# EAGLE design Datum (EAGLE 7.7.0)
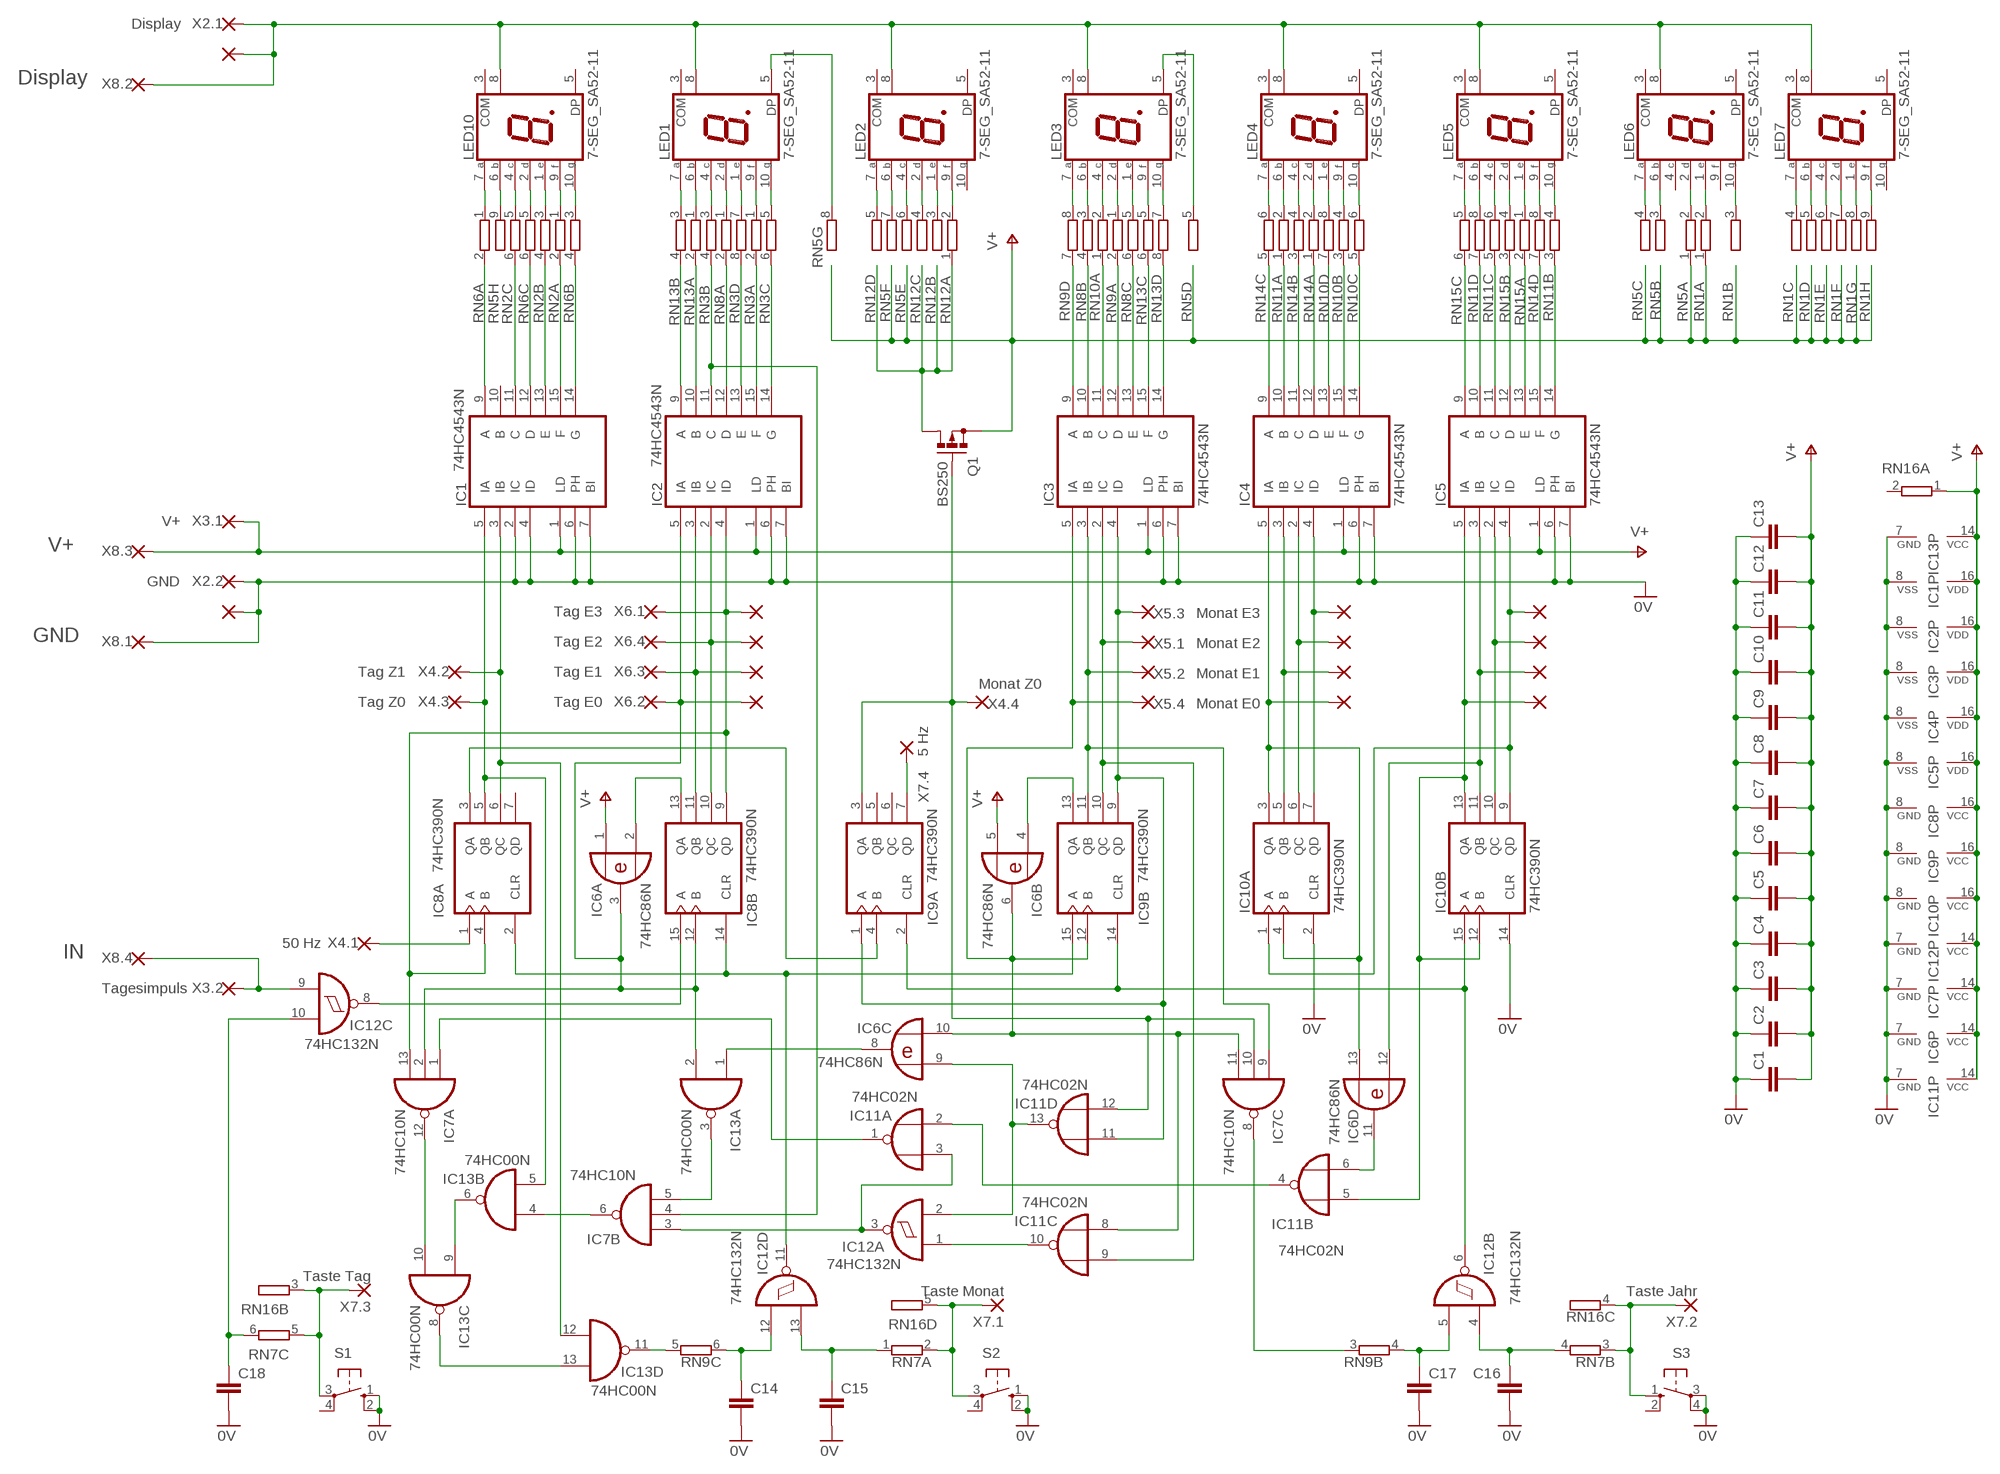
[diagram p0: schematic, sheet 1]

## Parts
102  WIREPAD1,6/0,8  [1,6/0,8]
104  WIREPAD1,6/0,8  [1,6/0,8]
111  WIREPAD1,6/0,8  [1,6/0,8]
112  WIREPAD1,6/0,8  [1,6/0,8]
113  Tag E0  WIREPAD1,6/0,8  [1,6/0,8]
114  WIREPAD1,6/0,8  [1,6/0,8]
119  WIREPAD1,6/0,8  [1,6/0,8]
120  WIREPAD1,6/0,8  [1,6/0,8]
121  WIREPAD1,6/0,8  [1,6/0,8]
122  WIREPAD1,6/0,8  [1,6/0,8]
123  WIREPAD1,6/0,8  [1,6/0,8]
124  WIREPAD1,6/0,8  [1,6/0,8]
125  WIREPAD1,6/0,8  [1,6/0,8]
126  WIREPAD1,6/0,8  [1,6/0,8]
C1  C-EU050-024X044  [C050-024X044]
C2  C-EU050-024X044  [C050-024X044]
C3  C-EU050-024X044  [C050-024X044]
C4  C-EU050-024X044  [C050-024X044]
C5  C-EU050-024X044  [C050-024X044]
C6  C-EU050-024X044  [C050-024X044]
C7  C-EU050-024X044  [C050-024X044]
C8  C-EU050-024X044  [C050-024X044]
C9  C-EU050-024X044  [C050-024X044]
C10  C-EU050-024X044  [C050-024X044]
C11  C-EU050-024X044  [C050-024X044]
C12  C-EU050-024X044  [C050-024X044]
C13  C-EU050-024X044  [C050-024X044]
C14  C-EU050-024X044  [C050-024X044]
C15  C-EU050-024X044  [C050-024X044]
C16  C-EU050-024X044  [C050-024X044]
C17  C-EU050-024X044  [C050-024X044]
C18  C-EU050-024X044  [C050-024X044]
IC1  74HC4543N  4543N  [DIL16]
IC2  74HC4543N  4543N  [DIL16]
IC3  74HC4543N  4543N  [DIL16]
IC4  74HC4543N  4543N  [DIL16]
IC5  74HC4543N  4543N  [DIL16]
IC6  74HC86N  [DIL14]
IC7  74HC10N  [DIL14]
IC8  74HC390N  [DIL16]
IC9  74HC390N  [DIL16]
IC10  74HC390N  [DIL16]
IC11  74HC02N  [DIL14]
IC12  74HC132N  [DIL14]
IC13  74HC00N  [DIL14]
LED1  7-SEG_SA52-11  [SA52-11]
LED2  7-SEG_SA52-11  [SA52-11]
LED3  7-SEG_SA52-11  [SA52-11]
LED4  7-SEG_SA52-11  [SA52-11]
LED5  7-SEG_SA52-11  [SA52-11]
LED6  7-SEG_SA52-11  [SA52-11]
LED7  7-SEG_SA52-11  [SA52-11]
LED10  7-SEG_SA52-11  [SA52-11]
Q1  BS250  [SOT54E]
RN1  GE08R  [SIL9]
RN2  E3R  [SIL6]
RN3  E4R  [SIL8]
RN5  GE08R  [SIL9]
RN6  E3R  [SIL6]
RN7  E3R  [SIL6]
RN8  E3R  [SIL6]
RN9  E4R  [SIL8]
RN10  E4R  [SIL8]
RN11  E4R  [SIL8]
RN12  GE04R  [SIL5]
RN13  E4R  [SIL8]
RN14  E4R  [SIL8]
RN15  E3R  [SIL6]
RN16  GE04R  [SIL5]
S1  10-XX  [B3F-10XX]
S2  10-XX  [B3F-10XX]
S3  10-XX  [B3F-10XX]
X2.1  Display  WIREPAD1,6/0,8  [1,6/0,8]
X2.2  GND  WIREPAD1,6/0,8  [1,6/0,8]
X3.1  V+  WIREPAD1,6/0,8  [1,6/0,8]
X3.2  Tagesimpuls  WIREPAD1,6/0,8  [1,6/0,8]
X4.1  50 Hz  WIREPAD1,6/0,8  [1,6/0,8]
X4.2  Tag Z1  WIREPAD1,6/0,8  [1,6/0,8]
X4.3  Tag Z0  WIREPAD1,6/0,8  [1,6/0,8]
X4.4  Monat Z0  WIREPAD1,6/0,8  [1,6/0,8]
X5.1  Monat E2  WIREPAD1,6/0,8  [1,6/0,8]
X5.2  Monat E1  WIREPAD1,6/0,8  [1,6/0,8]
X5.3  Monat E3  WIREPAD1,6/0,8  [1,6/0,8]
X5.4  Monat E0  WIREPAD1,6/0,8  [1,6/0,8]
X6.1  Tag E3  WIREPAD1,6/0,8  [1,6/0,8]
X6.2  Tag E0  WIREPAD1,6/0,8  [1,6/0,8]
X6.3  Tag E1  WIREPAD1,6/0,8  [1,6/0,8]
X6.4  Tag E2  WIREPAD1,6/0,8  [1,6/0,8]
X7.1  Taste Monat  WIREPAD1,6/0,8  [1,6/0,8]
X7.2  Taste Jahr  WIREPAD1,6/0,8  [1,6/0,8]
X7.3  Taste Tag  WIREPAD1,6/0,8  [1,6/0,8]
X7.4  5 Hz  WIREPAD1,6/0,8  [1,6/0,8]
X8.1  WIREPAD1,6/0,8  [1,6/0,8]
X8.2  WIREPAD1,6/0,8  [1,6/0,8]
X8.3  WIREPAD1,6/0,8  [1,6/0,8]
X8.4  WIREPAD1,6/0,8  [1,6/0,8]

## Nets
0V: 104.1(P) C1.1 C2.1 C3.1 C4.1 C5.1 C6.1 C7.1 C8.1 C9.1 C10.1 C11.1 C12.1 C13.1 C14.2 C15.2 C16.2 C17.2 C18.2 IC1.2(IC) IC1.4(ID) IC1.6(PH) IC1.7(BI) IC1.8(VSS) IC2.6(PH) IC2.7(BI) IC2.8(VSS) IC3.6(PH) IC3.7(BI) IC3.8(VSS) IC4.6(PH) IC4.7(BI) IC4.8(VSS) IC5.6(PH) IC5.7(BI) IC5.8(VSS) IC6.7(P:GND) IC7.7(P:GND) IC8.8(P:GND) IC9.8(P:GND) IC10.2(A:CLR) IC10.8(P:GND) IC10.14(B:CLR) IC11.7(P:GND) IC12.7(P:GND) IC13.7(P:GND) S1.1(S) S1.2(S1) S2.1(S) S2.2(S1) S3.3(P) S3.4(P1) X2.2.1(P) X8.1.1(P)
N$1: LED3.7(A) RN9.8
N$2: LED3.6(B) RN8.3
N$3: LED3.4(C) RN10.2
N$4: LED3.2(D) RN9.1
N$5: LED3.1(E) RN8.5
N$6: LED3.9(F) RN13.5
N$7: LED3.10(G) RN13.7
N$8: LED3.5(DP) RN5.5
N$9: LED1.5(DP) RN5.8
N$10: LED2.7(A) RN12.5
N$11: LED2.4(C) RN5.6
N$12: LED2.6(B) RN5.7
N$13: LED2.2(D) RN12.4
N$14: LED2.1(E) RN12.3
N$15: LED2.9(F) RN12.2
N$16: Q1.D RN12.1
N$17: IC6.2(A:I1) IC8.13(B:QA)
N$18: IC9.2(A:CLR) IC9.14(B:CLR) IC10.15(B:A) IC12.6(B:O)
N$19: LED6.7(A) RN5.4
N$20: IC3.9(A) RN9.7
N$21: IC3.10(B) RN8.4
N$22: LED5.4(C) RN11.6
N$23: IC3.12(D) RN9.2
N$24: IC3.13(E) RN8.6
N$25: IC3.15(F) RN13.6
N$26: IC3.14(G) RN13.8
N$27: LED4.7(A) RN14.6
N$28: LED4.6(B) RN11.2
N$29: LED4.4(C) RN14.4
N$30: LED4.2(D) RN14.2
N$31: LED4.1(E) RN10.8
N$32: LED4.9(F) RN10.4
N$33: LED4.10(G) RN10.6
N$34: LED5.7(A) RN15.5
N$35: LED5.6(B) RN11.8
N$36: IC4.10(B) RN11.1
N$37: LED5.2(D) RN15.4
N$38: LED5.1(E) RN15.1
N$39: LED5.9(F) RN14.8
N$40: LED5.10(G) RN11.4
N$41: IC5.14(G) RN11.3
N$42: IC5.15(F) RN14.7
N$43: IC5.13(E) RN15.2
N$44: IC5.12(D) RN15.3
N$45: IC2.15(F) RN3.2
N$46: IC5.10(B) RN11.7
N$47: IC5.9(A) RN15.6
N$48: IC4.14(G) RN10.5
N$49: IC4.15(F) RN10.3
N$50: IC4.13(E) RN10.7
N$51: IC4.12(D) RN14.1
N$52: IC4.11(C) RN14.3
N$54: IC4.9(A) RN14.5
N$55: LED6.6(B) RN5.3
N$56: LED6.2(D) RN5.2
N$57: LED6.1(E) RN1.2
N$58: LED6.10(G) RN1.3
N$59: LED7.7(A) RN1.4
N$60: LED7.6(B) RN1.5
N$61: LED7.4(C) RN1.6
N$62: LED7.2(D) RN1.7
N$63: LED7.1(E) RN1.8
N$64: LED7.9(F) RN1.9
N$65: IC5.11(C) RN11.5
N$66: 102.1(P) LED1.8(COM) LED2.8(COM) LED3.8(COM) LED4.8(COM) LED5.8(COM) LED6.8(COM) LED7.8(COM) LED10.8(COM) X2.1.1(P) X8.2.1(P)
N$67: 114.1(P) IC2.5(IA) IC6.3(A:O) IC7.2(A:I1) IC8.12(B:B) IC13.2(A:I1) X6.2.1(P)
N$68: IC11.2(A:I0) IC11.4(B:O)
N$69: 111.1(P) IC2.2(IC) IC8.10(B:QC) X6.4.1(P)
N$70: 113.1(P) IC2.4(ID) IC7.13(A:I2) IC8.4(A:B) IC8.9(B:QD) X6.1.1(P)
N$71: IC1.5(IA) IC8.5(A:QB) IC13.5(B:I1) X4.3.1(P)
N$72: IC1.3(IB) IC8.6(A:QC) IC13.12(D:I0) X4.2.1(P)
N$73: IC1.9(A) RN6.2
N$74: IC3.11(C) RN10.1
N$75: IC1.11(C) RN2.6
N$76: IC1.12(D) RN6.6
N$77: IC1.13(E) RN2.4
N$78: IC1.15(F) RN2.2
N$79: IC1.14(G) RN6.4
N$80: IC2.9(A) RN13.4
N$81: IC2.10(B) RN13.2
N$82: IC2.11(C) IC7.4(B:I1) RN3.4
N$83: IC2.12(D) RN8.2
N$84: IC2.13(E) RN3.8
N$86: IC2.14(G) RN3.6
N$87: LED1.10(G) RN3.5
N$88: LED1.9(F) RN3.1
N$89: LED1.1(E) RN3.7
N$90: LED1.2(D) RN8.1
N$91: LED1.4(C) RN3.3
N$92: LED1.6(B) RN13.1
N$93: LED1.7(A) RN13.3
N$94: LED10.10(G) RN6.3
N$95: LED10.9(F) RN2.1
N$96: LED10.1(E) RN2.3
N$97: LED10.2(D) RN6.5
N$98: LED10.4(C) RN2.5
N$99: LED10.6(B) RN5.9
N$100: LED10.7(A) RN6.1
N$101: IC6.4(B:I0) IC9.13(B:QA)
N$102: IC3.3(IB) IC7.9(C:I0) IC9.11(B:QB) X5.2.1(P)
N$103: IC3.2(IC) IC9.10(B:QC) IC11.9(C:I1) X5.1.1(P)
N$104: IC3.4(ID) IC9.1(A:A) IC9.9(B:QD) IC11.11(D:I0) X5.3.1(P)
N$105: 122.1(P) IC4.5(IA) IC6.13(D:I1) IC10.3(A:QA) IC10.4(A:B)
N$106: 120.1(P) IC4.3(IB) IC10.5(A:QB)
N$107: 119.1(P) IC4.2(IC) IC10.6(A:QC)
N$108: 121.1(P) IC4.4(ID) IC10.7(A:QD)
N$109: 126.1(P) IC5.5(IA) IC10.12(B:B) IC10.13(B:QA) IC11.5(B:I0)
N$110: 124.1(P) IC5.3(IB) IC6.12(D:I0) IC10.11(B:QB)
N$111: 123.1(P) IC5.2(IC) IC10.10(B:QC)
N$112: 125.1(P) IC5.4(ID) IC10.1(A:A) IC10.9(B:QD)
N$113: IC3.5(IA) IC6.6(B:O) IC6.10(C:I1) IC7.11(C:I2) IC9.12(B:B) IC11.8(C:I0) X5.4.1(P)
N$114: IC7.3(B:I0) IC11.3(A:I1) IC12.3(A:O)
N$115: IC7.5(B:I2) IC13.3(A:O)
N$116: IC7.1(A:I0) IC11.1(A:O)
N$117: IC6.8(C:O) IC13.1(A:I0)
N$118: IC7.12(A:O) IC13.10(C:I1)
N$119: IC13.6(B:O) IC13.9(C:I0)
N$120: IC7.6(B:O) IC13.4(B:I0)
N$121: IC13.8(C:O) IC13.13(D:I1)
N$122: IC8.2(A:CLR) IC8.14(B:CLR) IC9.15(B:A) IC12.11(D:O)
N$123: IC6.9(C:I0) IC11.13(D:O) IC12.2(A:I1)
N$124: IC11.10(C:O) IC12.1(A:I0)
N$125: IC12.9(C:I0) X3.2.1(P) X8.4.1(P)
N$126: 112.1(P) IC2.3(IB) IC8.11(B:QB) X6.3.1(P)
N$127: IC7.10(C:I1) IC9.3(A:QA) IC11.12(D:I1) Q1.G X4.4.1(P)
N$128: IC8.15(B:A) IC12.8(C:O)
N$129: IC6.11(D:O) IC11.6(B:I1)
N$131: IC13.11(D:O) RN9.5
N$132: C14.1 IC12.12(D:I0) RN9.6
N$133: RN7.2 RN16.5 S2.3(P) X7.1.1(P)
N$134: C15.1 IC12.13(D:I1) RN7.1
N$135: C17.1 IC12.5(B:I1) RN9.4
N$136: IC7.8(C:O) RN9.3
N$137: RN7.3 RN16.4 S3.1(S) X7.2.1(P)
N$138: C16.1 IC12.4(B:I0) RN7.4
N$139: C18.1 IC12.10(C:I1) RN7.6
N$140: RN7.5 RN16.3 S1.3(P) X7.3.1(P)
N$143: IC8.1(A:A) X4.1.1(P)
N$144: IC9.7(A:QD) X7.4.1(P)
N$145: IC8.3(A:QA) IC9.4(A:B)
V+: C1.2 C2.2 C3.2 C4.2 C5.2 C6.2 C7.2 C8.2 C9.2 C10.2 C11.2 C12.2 C13.2 IC1.1(LD) IC1.16(VDD) IC2.1(LD) IC2.16(VDD) IC3.1(LD) IC3.16(VDD) IC4.1(LD) IC4.16(VDD) IC5.1(LD) IC5.16(VDD) IC6.1(A:I0) IC6.5(B:I1) IC6.14(P:VCC) IC7.14(P:VCC) IC8.16(P:VCC) IC9.16(P:VCC) IC10.16(P:VCC) IC11.14(P:VCC) IC12.14(P:VCC) IC13.14(P:VCC) Q1.S RN1.1 RN5.1 RN16.1 X3.1.1(P) X8.3.1(P)
Unconnected: IC1.10(B) IC8.7(A:QD) IC9.5(A:QB) IC9.6(A:QC) LED1.3(COM) LED2.3(COM) LED2.5(DP) LED2.10(G) LED3.3(COM) LED4.3(COM) LED4.5(DP) LED5.3(COM) LED5.5(DP) LED6.3(COM) LED6.4(C) LED6.5(DP) LED6.9(F) LED7.3(COM) LED7.5(DP) LED7.10(G) LED10.3(COM) LED10.5(DP) RN16.2 S1.4(P1) S2.4(P1) S3.2(S1)

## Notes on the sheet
- Display
- V+
- GND
- IN

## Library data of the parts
102 104 111-114 119-126 X2.1 X2.2 X3.1 X3.2 X4.1-X4.4 X5.1-X5.4 X6.1-X6.4 X7.1-X7.4 X8.1-X8.4 = wirepad:WIREPAD: Wire PAD connect wire on PCB
C1-C18 = rclxrund:C-EU: CAPACITOR, European symbol; SPICEPREFIX: C
IC1-IC5 = 45xxrund:4543: BCD to 7-segment LCD DECODER
IC6 = 74xx-eu:74*86: Quad 2-input EXCLUSIVE-OR (XOR) gate
IC7 = 74xx-eu:74*10: Triple 3-input NAND gate
IC8-IC10 = 74xx-eu:74*390: Dual 4-bit decade and binary COUNTER
IC11 = 74xx-eu:74*02: Quad 2-input NOR gate
IC12 = 74xx-eu:74*132: Quad 2-input NAND schmitt trigger
IC13 = 74xx-eu:74*00: Quad 2-input NAND gate
LED1-LED7 LED10 = display-kingbrightyx:7-SEG_: Kingbright 14.2mm (0.56 INCH) SINGLE DIGIT NUMERIC DUISPLAY Source: SA56-11EWA(Ver1189471036.pdf; OC_FARNELL: unknown; OC_NEWARK: unknown
Q1 = transistor-small-signal:BS250: P-CHANNEL MOS FET
RN1 RN5 = resistor-silxrund:GE08R: SIL RESISTOR; OC_FARNELL: unknown; OC_NEWARK: unknown
RN2 RN6-RN8 RN15 = resistor-silxrund:E3R: SIL RESISTOR; OC_FARNELL: unknown; OC_NEWARK: unknown
RN3 RN9-RN11 RN13 RN14 = resistor-silxrund:E4R: SIL RESISTOR; OC_FARNELL: unknown; OC_NEWARK: unknown
RN12 RN16 = resistor-silxrund:GE04R: SIL RESISTOR; OC_FARNELL: unknown; OC_NEWARK: unknown
S1-S3 = switch-omronxrund:10-XX: OMRON SWITCH; MPN: B3F-1000; OC_FARNELL: 176432; OC_NEWARK: 36M3542

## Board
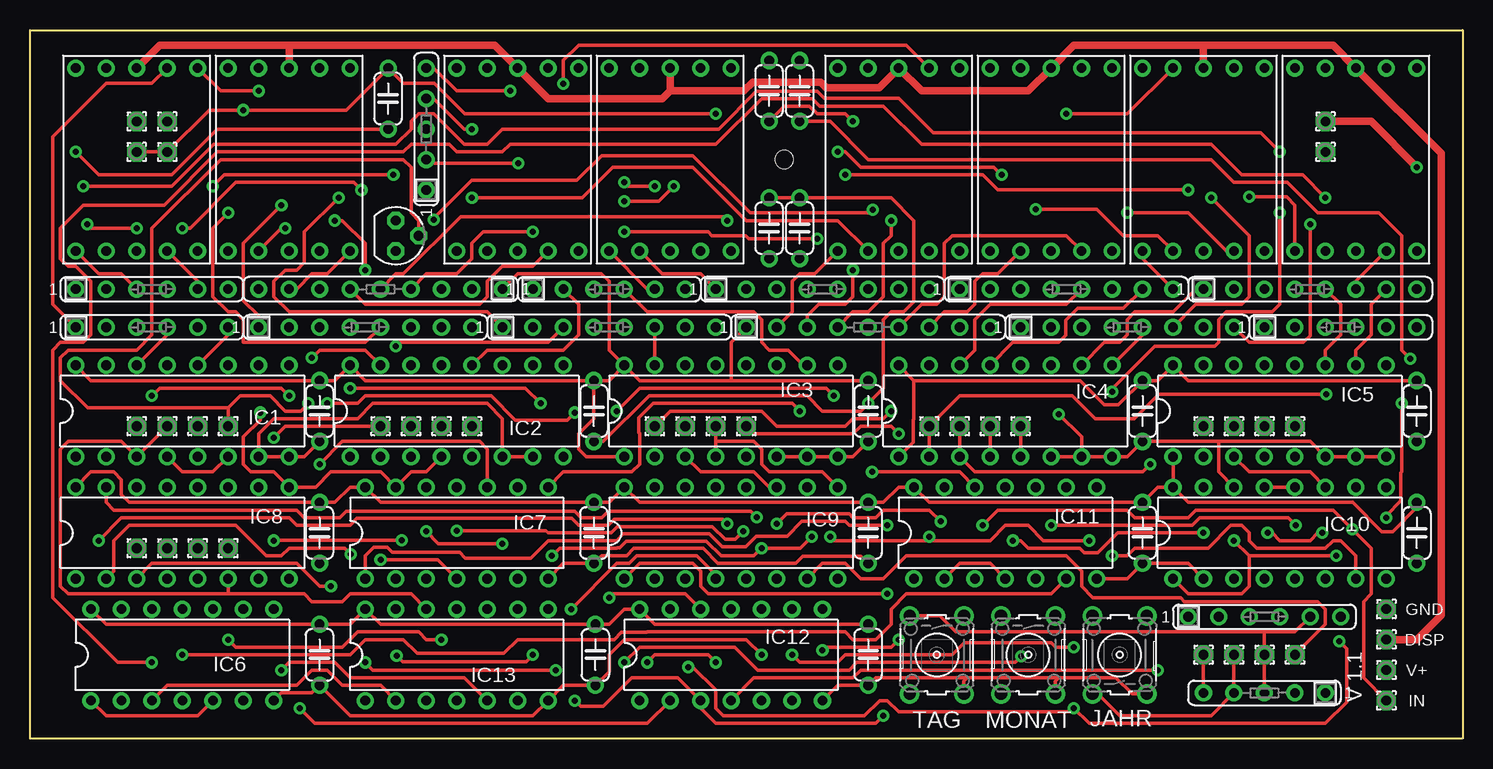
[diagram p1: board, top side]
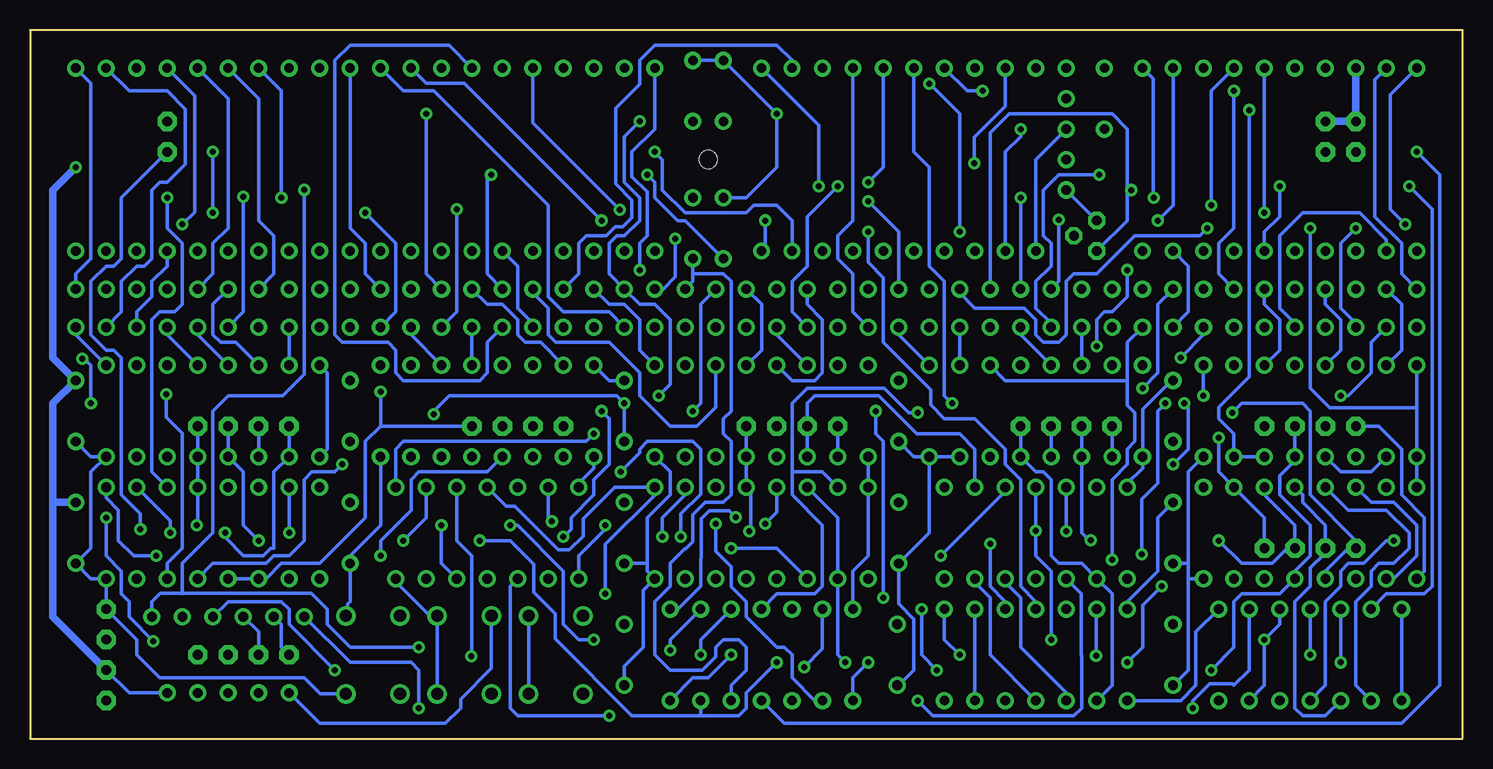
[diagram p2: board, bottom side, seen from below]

Size 119.38 x 59.05 mm. Coordinates in mm from the lower left corner, seen from the top.
Outline: 0,0 0,59.05 119.38,59.05 119.38,0 0,0
Copper layers (1*16): Top 0.035mm / dielectric 1.5mm / Bottom 0.035mm
Design rules "12mil *": minimum track width 12mil, minimum drill 0.5mm, track to track 12mil, track to pad 14mil, pad to pad 16mil, via to via 16mil, smd to smd 6mil, copper to edge 35mil, drill to drill 12mil, minimum pad ring 12mil, minimum via ring 10mil, stop-mask expansion 4mil, vias tented up to drill 0mil, thermal gap 10mil
Holes 1.5 mm at 62.87,48.26

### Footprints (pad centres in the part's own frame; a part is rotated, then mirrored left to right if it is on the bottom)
1,6/0,8 = drill 0.813 pad 1.6 octagon: 1 0,0
C050-024X044 = drill 0.813: 1 -2.54,0; 2 2.54,0
DIL16 = drill 0.813: 1 -8.89,-3.81; 2 -6.35,-3.81; 3 -3.81,-3.81; 4 -1.27,-3.81; 5 1.27,-3.81; 6 3.81,-3.81; 7 6.35,-3.81; 8 8.89,-3.81; 9 8.89,3.81; 10 6.35,3.81; 11 3.81,3.81; 12 1.27,3.81; 13 -1.27,3.81; 14 -3.81,3.81; 15 -6.35,3.81; 16 -8.89,3.81
DIL14 = drill 0.813: 1 -7.62,-3.81; 2 -5.08,-3.81; 3 -2.54,-3.81; 4 0,-3.81; 5 2.54,-3.81; 6 5.08,-3.81; 7 7.62,-3.81; 8 7.62,3.81; 9 5.08,3.81; 10 2.54,3.81; 11 0,3.81; 12 -2.54,3.81; 13 -5.08,3.81; 14 -7.62,3.81
SA52-11 = drill 0.8: 1 -5.08,-7.62; 2 -2.54,-7.62; 3 0,-7.62; 4 2.54,-7.62; 5 5.08,-7.62; 6 5.08,7.62; 7 2.54,7.62; 8 0,7.62; 9 -2.54,7.62; 10 -5.08,7.62
SOT54E = drill 0.813 octagon: D -1.27,0; G 0,1.905; S 1.27,0
SIL9 = drill 0.813: 1 -10.16,0; 2 -7.62,0; 3 -5.08,0; 4 -2.54,0; 5 0,0; 6 2.54,0; 7 5.08,0; 8 7.62,0; 9 10.16,0
SIL6 = drill 0.813: 1 -6.35,0; 2 -3.81,0; 3 -1.27,0; 4 1.27,0; 5 3.81,0; 6 6.35,0
SIL8 = drill 0.813: 1 -8.89,0; 2 -6.35,0; 3 -3.81,0; 4 -1.27,0; 5 1.27,0; 6 3.81,0; 7 6.35,0; 8 8.89,0
SIL5 = drill 0.813: 1 -5.08,0; 2 -2.54,0; 3 0,0; 4 2.54,0; 5 5.08,0
B3F-10XX = drill 1.016: 1 -3.251,2.261; 2 3.251,2.261; 3 -3.251,-2.261; 4 3.251,-2.261

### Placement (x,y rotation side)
102  11.43,51.44 0 top
104  11.43,48.9 0 top
111  29.21,26.04 0 top
112  31.75,26.04 0 top
113  34.29,26.04 0 top
114  36.83,26.04 0 top
119  74.93,26.04 0 top
120  77.47,26.04 0 top
121  80.01,26.04 0 top
122  82.55,26.04 0 top
123  97.79,26.04 0 top
124  100.33,26.04 0 top
125  102.87,26.04 0 top
126  105.41,26.04 0 top
C1  115.57,27.3 90 top
C2  24.13,27.3 90 top
C3  46.99,27.3 90 top
C4  69.85,27.3 90 top
C5  92.71,27.3 90 top
C6  115.57,17.14 90 top
C7  24.13,17.14 90 top
C8  69.85,6.99 90 top
C9  24.13,6.99 90 top
C10  92.71,17.14 90 top
C11  69.85,17.14 90 top
C12  46.99,17.14 90 top
C13  47.12,6.99 90 top
C14  61.59,53.98 90 top
C15  64.14,53.98 90 top
C16  29.84,53.34 90 top
C17  64.14,42.55 90 top
C18  61.59,42.55 90 top
IC1  12.7,27.3 0 top
IC2  35.56,27.3 0 top
IC3  58.42,27.3 0 top
IC4  81.28,27.3 0 top
IC5  104.14,27.3 0 top
IC6  12.7,6.99 0 top
IC7  35.56,17.14 0 top
IC8  12.7,17.14 0 top
IC9  58.42,17.14 0 top
IC10  104.14,17.14 0 top
IC11  81.28,17.14 0 top
IC12  58.42,6.99 0 top
IC13  35.56,6.99 0 top
LED1  21.59,48.26 0 top
LED2  40.64,48.26 0 top
LED3  53.34,48.26 0 top
LED4  97.79,48.26 0 top
LED5  110.49,48.26 0 top
LED6  72.39,48.26 0 top
LED7  85.09,48.26 0 top
LED10  8.89,48.26 0 top
Q1  30.48,41.91 270 top
RN1  69.85,34.29 0 top
RN2  10.16,37.47 0 top
RN3  27.94,34.29 0 top
RN5  29.21,37.47 180 top
RN6  10.16,34.29 0 top
RN7  102.87,10.16 0 top
RN8  48.26,37.47 0 top
RN9  66.04,37.47 0 top
RN10  86.36,37.47 0 top
RN11  106.68,37.47 0 top
RN12  33.02,50.8 90 top
RN13  48.26,34.29 0 top
RN14  91.44,34.29 0 top
RN15  109.22,34.29 0 top
RN16  102.87,3.81 180 top
S1  75.56,6.99 270 top
S2  83.19,6.99 270 top
S3  90.81,6.99 90 top
X2.1  8.89,51.44 0 top
X2.2  8.89,48.9 0 top
X3.1  107.95,51.44 0 top
X3.2  107.95,48.9 0 top
X4.1  8.89,26.04 0 top
X4.2  11.43,26.04 0 top
X4.3  13.97,26.04 0 top
X4.4  16.51,26.04 0 top
X5.1  52.07,26.04 0 top
X5.2  54.61,26.04 0 top
X5.3  57.15,26.04 0 top
X5.4  59.69,26.04 0 top
X6.1  8.89,15.88 0 top
X6.2  11.43,15.88 0 top
X6.3  13.97,15.88 0 top
X6.4  16.51,15.88 0 top
X7.1  97.79,6.99 0 top
X7.2  100.33,6.99 0 top
X7.3  102.87,6.99 0 top
X7.4  105.41,6.99 0 top
X8.1  113.03,10.79 0 top
X8.2  113.03,8.26 0 top
X8.3  113.03,5.71 0 top
X8.4  113.03,3.17 0 top

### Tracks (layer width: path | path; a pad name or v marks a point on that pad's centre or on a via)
0V  (via drill 0.5)
  Top 0.305: IC5.8 IC5.7 IC5.6 106.68,24.77 99.06,24.77 | IC4.7 IC4.6 | IC4.7 IC4.8 91.44,23.5 C5.1 99.06,24.77 | IC10.14 99.06,22.23 99.06,24.77 | IC3.6 IC3.7 IC3.8 68.58,23.5 C4.1 | IC12.7 67.31,4.45 C8.1 70.48,5.08 78.11,5.08 | IC11.7 91.44,13.34 C10.1 96.52,14.61 IC10.2 | 85.72,5.08 90.49,5.08 91.83,3.73 S3.3 | S2.2 85.45,4.8 85.72,5.08 | C18.2 C17.2 71.75,45.09 73.66,43.18 73.66,36.42 72.8,35.56 71.75,35.56 71.12,34.92 71.12,29.21 v69.85,27.94 69.22,27.3 66.04,27.3 64.77,28.57 51.6,28.57 47.79,24.77 C3.1 | IC7.7 44.45,14.61 C12.1 47.62,15.24 49.71,15.24 50.32,15.85 56.11,15.85 57.33,14.63 63.82,14.63 64.4,15.21 69.24,15.21 C11.1 | IC2.7 IC2.6 39.37,26.67 38.1,27.94 28.57,27.94 27.3,26.67 20.32,26.67 19.05,25.4 IC1.7 IC1.8 22.86,23.5 C2.1 | IC6.7 20.95,3.81 23.5,3.81 C9.1 26.67,1.91 41.91,1.91 IC13.7 44.45,4.45 C13.1 48.26,5.59 48.26,6.99 49.53,8.26 59.69,8.26 v60.96,6.99 | IC1.4 12.7,22.23 15.24,22.23 IC1.6 | v85.72,27.05 87.63,25.14 IC4.7 | 85.72,5.08 78.11,5.08 | S1.2 77.83,4.8 78.11,5.08 | v57.15,52.07 36.22,52.07 33.68,54.61 31.11,54.61 C16.2 26.35,52.39 v17.78,52.39 14.92,52.39 104.1 X2.2.1
  Bottom 0.305: 67.94,14.61 67.94,13.97 IC9.8 68.26,12.38 68.26,7.62 69.85,6.03 C8.1 | C11.1 67.94,14.61 | IC3.8 66.04,22.23 66.04,20.32 67.94,18.41 67.94,14.61 | IC11.7 88.9,13.06 86.08,10.24 S2.1 S2.2 | S3.4 92.91,11.23 92.71,11.43 C10.1 92.71,15.24 90.17,17.78 IC4.8 | IC2.7 IC2.8 | C3.1 45.72,23.5 IC2.8 | IC2.8 44.45,17.14 C12.1 46.99,11.24 45.72,9.97 45.72,5.71 46.99,4.45 C13.1 | 22.86,13.34 IC8.8 | 22.86,13.34 22.86,5.71 C9.1 | IC1.6 IC1.7 19.05,25.4 20.32,26.67 20.32,27.62 17.78,30.16 v17.78,52.39 | 22.86,14.61 22.86,22.23 IC1.8 | IC12.7 64.14,5.08 62.87,5.08 v60.96,6.99 | IC1.4 10.16,22.23 7.62,22.23 IC1.2 | C1.1 114.3,23.5 IC5.8 114.3,22.23 114.3,15.88 C6.1 114.3,13.34 IC10.8 X8.1.1 110.49,8.26 110.49,6.99 108.58,5.08 96.52,5.08 95.17,3.73 S3.3 | C4.1 v69.85,27.94 70.48,28.57 84.45,28.57 85.72,27.3 v85.72,27.05 | S1.1 S1.2 | 22.86,14.61 22.86,13.34 | C7.1 22.86,14.61 | C15.2 C14.2 v57.15,52.07 57.15,47.62 59.69,45.09 C18.2
N$1
  Bottom 0.305: RN9.8 73.66,38.73 73.66,41.27 73.03,41.91 71.37,41.91 70.61,42.67 69.98,42.67 69.96,42.66 69.22,43.41 69.22,44.86 70.58,46.22 70.58,52.55 68.58,54.55 68.58,56.52 67.31,57.78 57.15,57.78 55.88,56.52 LED3.7
N$2  (via drill 0.5)
  Top 0.305: v53.66,46.04 52.39,44.77 v49.53,44.77
  Bottom 0.305: v53.66,46.04 53.66,51.12 LED3.6 | v49.53,44.77 46.99,42.23 RN8.3
N$3  (via drill 0.5)
  Top 0.305: v67.31,48.9 67.94,48.9 69.22,47.62 80.33,47.62 v80.96,46.99
  Bottom 0.305: v67.31,48.9 66.67,48.26 66.67,45.72 64.77,43.81 59.69,43.81 59.05,44.45 57.15,44.45 55.88,43.18 LED3.4 | v80.96,46.99 81.28,46.67 81.28,38.73 RN10.2
N$4
  Top 0.305: LED3.2 52.7,38.73 55.88,38.73 RN9.1
N$5
  Top 0.305: LED3.1 51.44,37.47 RN8.5
N$6
  Bottom 0.305: LED3.9 50.8,43.18 52.07,41.91 52.07,40.01 50.8,38.73 50.8,35.56 RN13.5
N$7  (via drill 0.5)
  Top 0.305: v49.53,46.35 49.85,46.04 v52.07,46.04
  Bottom 0.305: v49.53,46.35 48.26,47.62 LED3.10 | v52.07,46.04 54.61,43.5 54.61,39.37 55.88,38.1 55.88,35.56 RN13.7
N$8  (via drill 0.5)
  Top 0.305: v58.1,43.18 57.78,43.5 35.88,43.5 31.11,38.73 30.48,38.73 RN5.5
  Bottom 0.305: LED3.5 58.1,40.96 v58.1,43.18
N$9
  Top 0.305: LED1.5 24.77,38.73 23.5,38.73 22.23,37.47 RN5.8
N$10  (via drill 0.5)
  Top 0.305: RN12.5 33.66,55.88 35.56,53.98 v40.01,53.98
  Bottom 0.305: LED2.7 41.27,53.98 v40.01,53.98
N$11
  Top 0.305: LED2.4 41.91,39.37 39.37,39.37 38.1,38.1 38.1,36.83 37.47,36.2 27.94,36.2 RN5.6
N$12  (via drill 0.5)
  Top 0.305: v42.55,27.94 41.27,29.21 v26.67,29.21
  Bottom 0.305: LED2.6 45.72,48.9 44.45,47.62 44.45,39.37 43.18,38.1 43.18,28.57 v42.55,27.94 | v26.67,29.21 25.4,30.48 25.4,36.2 RN5.7
N$13  (via drill 0.5)
  Top 0.305: v36.83,50.8 36.2,50.8 33.66,53.34 RN12.4
  Bottom 0.305: LED2.2 38.1,48.9 36.83,50.16 v36.83,50.8
N$14
  Bottom 0.305: LED2.1 35.56,48.26 RN12.3
N$15  (via drill 0.5)
  Top 0.305: v40.7,47.94 33.34,47.94 RN12.2
  Bottom 0.305: LED2.9 38.1,52.7 40.7,50.1 v40.7,47.94
N$16
  Bottom 0.305: RN12.1 Q1.D
N$17
  Bottom 0.305: IC6.2 8.89,4.45 8.89,11.43 7.62,12.7 7.62,13.97 6.99,14.61 5.71,14.61 4.45,15.88 4.45,17.14 6.35,19.05 9.53,19.05 IC8.13
N$18  (via drill 0.5)
  Top 0.305: v51.44,6.35 52.07,6.99 56.52,6.99 v57.15,6.35 | v81.92,16.51 82.55,16.51 83.19,15.88 87.47,15.88 87.85,15.5 89,15.5 90.64,17.14 v97.79,17.14
  Bottom 0.305: 63.5,1.91 60.33,1.91 59.69,2.54 59.69,3.81 v57.15,6.35 | IC9.14 52.07,18.41 IC9.2 52.07,6.99 v51.44,6.35 | v97.79,17.14 IC10.15 | 63.5,1.91 69.22,1.91 75.63,8.32 75.63,10.4 77.42,12.2 77.42,14.55 79.38,16.51 v81.92,16.51 | IC12.6 63.5,1.91
N$19  (via drill 0.5)
  Top 0.305: LED6.7 73.03,57.78 45.72,57.78 44.45,56.52 v44.45,54.58 | v41.91,42.23 37.78,42.23 36.83,41.27 36.83,40.01 35.56,38.73 33.02,38.73 RN5.4
  Bottom 0.305: v41.91,42.23 41.91,52.07 44.45,54.61 v44.45,54.58
N$20
  Bottom 0.305: IC3.9 68.58,32.38 68.58,34.92 69.85,36.2 71.12,36.2 RN9.7
N$21
  Top 0.305: RN8.4 51.44,35.56 60.33,35.56 60.96,34.92 60.96,33.02 61.59,32.38 63.18,32.38 64.45,31.11 IC3.10
N$22
  Top 0.305: LED5.4 110.49,38.1 RN11.6
N$23
  Bottom 0.305: IC3.12 58.42,32.38 58.42,36.2 RN9.2
N$24
  Bottom 0.305: RN8.6 54.61,36.2 53.34,34.92 53.34,30.48 53.98,29.84 55.88,29.84 IC3.13
N$25
  Top 0.305: RN13.6 IC3.15
N$26
  Bottom 0.305: IC3.14 57.15,33.66 RN13.8
N$27  (via drill 0.5)
  Top 0.305: RN14.6 97.16,36.2 100.97,36.2 101.6,36.83 101.6,41.91 v98.42,45.09
  Bottom 0.305: v98.42,45.09 98.42,53.98 LED4.7
N$28
  Bottom 0.305: RN11.2 99.06,38.73 99.06,41.91 100.33,43.18 100.33,53.34 LED4.6
N$29  (via drill 0.5)
  Top 0.305: v91.44,43.81 96.52,43.81 99.69,40.64 LED4.4
  Bottom 0.305: v91.44,43.81 88.9,41.27 88.9,35.56 RN14.4
N$30  (via drill 0.5)
  Top 0.305: LED4.2 93.98,41.91 91.12,41.91 88.9,44.13 v83.82,44.13
  Bottom 0.305: v83.82,44.13 83.82,35.56 RN14.2
N$31
  Top 0.305: RN10.8 92.71,40.01 LED4.1
N$32  (via drill 0.5)
  Top 0.305: LED4.9 91.44,52.07 v86.36,52.07
  Bottom 0.305: v86.36,52.07 86.36,38.73 RN10.4
N$33
  Bottom 0.305: LED4.10 92.71,42.55 91.44,41.27 91.44,38.73 RN10.6
N$34
  Bottom 0.305: LED5.7 111.12,53.98 107.95,53.98 106.43,52.45 106.43,47.88 107.95,46.35 108.58,46.35 109.22,45.72 109.22,40.01 109.86,39.37 110.49,39.37 111.76,38.1 111.76,35.56 RN15.5
N$35
  Bottom 0.305: LED5.6 114.3,54.61 114.3,40.01 115.57,38.73 RN11.8
N$36
  Top 0.305: IC4.10 89.53,33.02 90.81,33.02 91.44,33.66 91.44,34.92 92.08,35.56 95.25,35.56 97.16,37.47 RN11.1
N$37
  Bottom 0.305: RN15.4 110.49,35.56 109.22,36.83 109.22,38.1 107.95,39.37 LED5.2
N$38  (via drill 0.5)
  Top 0.305: LED5.1 105.41,44.45 104.71,45.15 v101.6,45.15
  Bottom 0.305: v101.6,45.15 101.6,35.56 RN15.1
N$39  (via drill 0.5)
  Top 0.305: v106.68,42.86 106.68,33.59 106.11,33.02 101.6,33.02 RN14.8
  Bottom 0.305: v106.68,42.86 105.66,43.88 105.66,53.59 LED5.9
N$40
  Bottom 0.305: RN11.4 104.14,38.73 104.14,41.27 102.87,42.55 102.87,53.34 LED5.10
N$41
  Bottom 0.305: IC5.14 102.23,33.02 103.5,33.02 104.14,33.66 104.14,36.2 RN11.3
N$42
  Bottom 0.305: RN14.7 IC5.15
N$43
  Bottom 0.305: IC5.13 105.41,33.66 RN15.2
N$44
  Bottom 0.305: IC5.12 107.95,33.66 RN15.3
N$45  (via drill 0.5)
  Top 0.305: IC2.15 27.94,32.38 24.13,32.38 v23.5,31.75
  Bottom 0.305: v23.5,31.75 21.59,33.66 RN3.2
N$46
  Top 0.305: IC5.10 110.49,32.38 111.76,33.66 111.76,36.2 RN11.7
N$47
  Bottom 0.305: IC5.9 115.57,33.66 RN15.6
N$48
  Top 0.305: IC4.14 78.74,32.38 78.74,34.92 80.01,36.2 86.36,36.2 RN10.5
N$49
  Bottom 0.305: IC4.15 76.83,33.02 78.11,33.02 78.74,33.66 78.74,34.92 80.01,36.2 81.28,36.2 RN10.3
N$50
  Top 0.305: IC4.13 81.92,33.02 85.72,33.02 86.31,33.6 86.31,34.87 87.31,35.88 91.12,35.88 RN10.7
N$51
  Bottom 0.305: RN14.1 IC4.12
N$52
  Bottom 0.305: IC4.11 87.63,33.66 RN14.3
N$54
  Top 0.305: IC4.9 92.71,33.66 RN14.5
N$55  (via drill 0.5)
  Top 0.305: v70.23,44.07 69.98,43.81 60.01,43.81 55.24,48.58 47.62,48.58 45.56,46.51 36.8,46.51 33.66,43.37 v33.66,43.24
  Bottom 0.305: LED6.6 77.47,51.31 v70.23,44.07 | v33.66,43.24 33.66,38.1 RN5.3
N$56  (via drill 0.5)
  Top 0.305: LED6.2 67.31,43.18 59.69,43.18 55.24,47.62 48.58,47.62 46.04,45.09 v36.83,45.09
  Bottom 0.305: RN5.2 v36.83,45.09
N$57
  Top 0.305: LED6.1 65.41,38.73 64.14,38.73 63.5,38.1 63.5,35.56 RN1.2
N$58  (via drill 0.5)
  Top 0.305: RN1.3 64.77,35.24 65.72,36.2 67.94,36.2 68.58,36.83 v68.58,39.05
  Bottom 0.305: LED6.10 67.31,50.8 69.22,48.9 69.22,46.83 67.94,45.56 67.94,41.91 68.58,41.27 v68.58,39.05
N$59  (via drill 0.5)
  Top 0.305: v71.75,43.18 71.75,41.91 71.12,41.27 71.12,36.83 69.85,35.56 68.58,35.56 RN1.4
  Bottom 0.305: LED7.7 86.36,54.61 83.19,54.61 v71.75,43.18
N$60
  Bottom 0.305: LED7.6 88.27,53.98 85.72,53.98 76.2,44.45 76.2,36.83 74.93,35.56 71.12,35.56 RN1.5
N$61
  Top 0.305: LED7.4 86.36,41.91 76.83,41.91 76.2,41.27 76.2,36.83 75.56,36.2 74.3,36.2 RN1.6
N$62
  Top 0.305: LED7.2 80.64,38.73 79.38,38.73 78.74,38.1 78.74,36.2 78.11,35.56 76.2,35.56 RN1.7
N$63
  Bottom 0.305: LED7.1 78.74,39.37 78.74,35.88 77.47,34.61 RN1.8
N$64
  Bottom 0.305: LED7.9 84.45,57.78 92.71,57.78 93.98,56.52 93.98,33.66 93.34,33.02 89.53,33.02 88.9,32.38 88.9,30.48 88.27,29.84 81.92,29.84 81.28,30.48 81.28,33.02 RN1.9
N$65
  Top 0.305: IC5.11 107.95,32.38 109.22,33.66 109.22,36.2 RN11.5
N$66
  Top 0.61: X8.2.1 115.57,8.26 117.6,10.29 117.6,48.77 LED5.8 108.58,57.78 97.79,57.78 | 97.79,57.78 87,57.78 LED7.8 83.19,53.98 74.3,53.98 LED6.8 70.77,54.26 66.35,54.26 65.9,54.71 60.21,54.71 59.47,53.98 53.34,53.98 | LED4.8 97.79,57.78 | 53.34,53.98 52.7,53.34 43.18,53.34 LED2.8 38.73,57.78 21.59,57.78 | 53.34,53.98 LED3.8 | 21.59,57.78 10.79,57.78 LED10.8 | LED1.8 21.59,57.78
  Bottom 0.61: LED10.8 X2.1.1 102.1
N$67
  Top 0.305: IC13.2 29.21,4.45 26.04,4.45 24.77,5.71 23.5,5.71 22.23,4.45 11.43,4.45 IC6.3
  Bottom 0.305: 114.1 IC2.5 35.56,22.23 34.92,22.23 34.29,21.59 34.29,15.24 33.66,14.61 31.75,14.61 IC7.2 29.21,12.06 29.21,4.45 IC13.2 | IC8.12 13.34,20.32 13.34,19.68 11.43,17.78 X6.2.1 11.43,15.47 12.68,14.22 12.68,13.99 12.7,13.97 12.7,12.7 13.97,11.43 13.97,2.54 13.34,1.91 11.43,1.91 IC6.3
N$68
  Top 0.305: IC11.2 77.47,14.61 80.01,14.61 IC11.4
N$69  (via drill 0.5)
  Top 0.305: v20.32,25.08 21.27,26.04 111.1
  Bottom 0.305: v20.32,25.08 20.32,22.23 IC8.10 16.51,18.41 X6.4.1 | 111.1 IC2.2
N$70  (via drill 0.5)
  Top 0.305: IC2.4 33.02,22.23 31.75,22.23 IC7.13 29.21,22.23 25.08,22.23 23.81,20.95 IC8.9 20.32,22.23 18.41,22.23 17.78,22.86 17.78,25.15 19.18,26.54 v19.18,27.18
  Bottom 0.305: IC2.4 113.1 | v19.18,27.18 18.41,27.94 13.34,27.94 12.7,27.3 12.7,20.32 8.89,16.51 X6.1.1 9.53,15.88 11.43,13.97 IC8.4
N$71  (via drill 0.5)
  Top 0.305: IC13.5 36.2,5.08 26.67,5.08 25.4,6.35 21.59,6.35 v20.95,5.71
  Bottom 0.305: v20.95,5.71 19.05,7.62 19.05,11.43 18.41,12.06 15.24,12.06 IC8.5 13.97,13.97 12.7,15.24 12.7,17.78 15.24,20.32 15.24,21.91 13.97,23.18 IC1.5 X4.3.1
N$72
  Top 0.305: X4.2.1 IC1.3 7.62,24.77 3.17,24.77 2.54,24.13 2.54,12.7 3.17,12.06 16.51,12.06 | 16.51,12.06 IC8.6 | 16.51,12.06 22.86,12.06 23.5,11.43 26.04,11.43 26.67,12.06 31.75,12.06 IC13.12
N$73  (via drill 0.5)
  Top 0.305: v21.59,28.57 20.95,29.21 10.79,29.21 v10.16,28.57
  Bottom 0.305: RN6.2 7.62,33.02 7.62,30.48 9.53,28.57 v10.16,28.57 | IC1.9 v21.59,28.57
N$74
  Bottom 0.305: IC3.11 62.23,27.62 63.82,26.04 66.04,26.04 68.58,28.57 68.58,30.48 71.12,33.02 75.56,33.02 76.2,33.66 76.2,35.88 77.47,37.15 RN10.1
N$75
  Bottom 0.305: IC1.11 15.24,32.38 15.24,34.92 16.51,36.2 RN2.6
N$76
  Top 0.305: IC1.12 16.51,33.66 RN6.6
N$77
  Bottom 0.305: IC1.13 10.16,32.38 10.16,34.92 11.43,36.2 RN2.4
N$78
  Bottom 0.305: IC1.15 5.08,32.38 5.08,36.2 RN2.2
N$79
  Top 0.305: IC1.14 11.43,33.66 RN6.4
N$80
  Bottom 0.305: IC2.9 46.99,33.66 RN13.4
N$81
  Bottom 0.305: RN13.2 IC2.10
N$82  (via drill 0.5)
  Top 0.305: IC7.4 33.97,14.92 v29.21,14.92
  Bottom 0.305: v29.21,14.92 29.21,21.59 27.94,22.86 27.94,24.13 27.3,24.77 27.3,27.14 27.94,27.78 27.94,29.84 | 27.94,29.84 27.94,33.02 RN3.4 | IC2.11 38.1,29.84 27.94,29.84
N$83
  Top 0.305: IC2.12 38.1,32.38 44.45,32.38 45.72,33.66 45.72,36.2 RN8.2
N$84
  Bottom 0.305: RN3.8 36.83,33.66 IC2.13
N$86
  Bottom 0.305: RN3.6 IC2.14
N$87  (via drill 0.5)
  Top 0.305: v16.51,43.81 15.24,42.55 15.24,36.83 16.51,35.56 17.14,35.56 17.78,34.92 17.78,33.02 27.94,33.02 RN3.5
  Bottom 0.305: v16.51,43.81 LED1.10
N$88  (via drill 0.5)
  Top 0.305: v20.95,44.45 17.78,41.27 17.78,36.51 19.05,35.24 RN3.1
  Bottom 0.305: LED1.9 20.95,53.98 v20.95,44.45
N$89  (via drill 0.5)
  Top 0.305: v15.24,46.04 16.19,46.99 v30.29,46.99
  Bottom 0.305: LED1.1 16.51,42.23 15.24,43.5 v15.24,46.04 | v30.29,46.99 33.66,46.99 34.92,45.72 34.92,41.91 34.29,41.27 34.29,39.37 35.56,38.1 35.56,35.88 34.29,34.61 RN3.7
N$90  (via drill 0.5)
  Top 0.305: LED1.2 20.95,42.55 v21.27,42.55
  Bottom 0.305: v21.27,42.55 21.91,41.91 27.3,41.91 30.48,38.73 32.38,38.73 33.02,38.1 33.02,33.66 33.66,33.02 34.92,33.02 35.56,33.66 35.56,34.92 36.51,35.88 40.64,35.88 41.91,37.15 RN8.1
N$91
  Bottom 0.305: LED1.4 22.86,39.37 22.86,35.56 RN3.3
N$92  (via drill 0.5)
  Top 0.305: v25.72,45.09 22.86,42.23 22.86,39.69 22.23,39.05 21.27,39.05 20.32,38.1 20.32,36.83 21.59,35.56 38.1,35.56 RN13.1
  Bottom 0.305: LED1.6 25.78,54.99 25.78,45.15 v25.72,45.09
N$93  (via drill 0.5)
  Top 0.305: v25.4,43.18 26.04,43.18 27.94,41.27 v27.94,39.05 | v30.48,32.7 30.8,33.02 43.18,33.02 RN13.3
  Bottom 0.305: LED1.7 24.13,44.45 v25.4,43.18 | v27.94,39.05 27.94,36.83 29.21,35.56 29.84,35.56 30.48,34.92 v30.48,32.7
N$94  (via drill 0.5)
  Top 0.305: v8.89,42.55 5.08,42.55 v4.76,42.86
  Bottom 0.305: LED10.10 6.03,53.66 6.03,44.13 v4.76,42.86 | v8.89,42.55 10.16,41.27 10.16,35.88 8.89,34.61 RN6.3
N$95
  Bottom 0.305: LED10.9 7.3,54.93 7.3,43.5 5.08,41.27 5.08,38.73 RN2.1
N$96
  Top 0.305: LED10.1 5.71,38.73 7.62,38.73 RN2.3
N$97
  Bottom 0.305: LED10.2 6.35,41.59 8.57,43.81 13.34,43.81 15.24,41.91 15.24,35.88 13.97,34.61 RN6.5
N$98
  Top 0.305: LED10.4 13.97,38.1 RN2.5
N$99  (via drill 0.5)
  Top 0.305: LED10.6 15.88,53.98 v19.05,53.98
  Bottom 0.305: v19.05,53.98 19.05,42.55 20.32,41.27 20.32,38.73 RN5.9
N$100
  Top 0.305: LED10.7 10.16,54.61 6.35,54.61 1.91,50.16 1.91,36.2 RN6.1
N$101  (via drill 0.5)
  Top 0.305: v5.71,16.51 7.62,18.41 21.59,18.41 22.23,17.78 26.67,17.78 27.24,18.35 45.15,18.35 45.72,17.78 48.2,17.78 48.7,18.29 57.72,18.29 v58.1,17.91
  Bottom 0.305: IC6.4 11.43,4.45 11.43,11.43 10.16,12.7 10.16,13.97 9.53,14.61 8.26,14.61 6.35,16.51 v5.71,16.51 | v58.1,17.91 57.15,18.86 IC9.13
N$102
  Top 0.305: IC9.11 61.59,20.95 60.33,22.23 55.88,22.23 IC3.3
  Bottom 0.305: IC7.9 40.64,24.13 41.91,25.4 45.47,25.4 48.64,28.57 53.98,28.57 54.61,27.94 X5.2.1 IC3.3
N$103  (via drill 0.5)
  Top 0.305: v66.67,16.83 66.99,16.51 74.93,16.51 | v71.75,27.3 71.12,26.67 68.58,26.67 67.94,26.04 62.23,26.04 60.96,27.3 53.34,27.3 X5.1.1 | 74.93,16.51 v74.93,16.83 | 74.93,16.51 80.01,16.51 81.28,17.78 83.19,17.78 84.45,16.51 v88.27,16.51
  Bottom 0.305: X5.1.1 IC3.2 | IC9.10 64.77,20.32 66.67,18.41 v66.67,16.83 | v88.27,16.51 86.36,18.41 IC11.9 | v71.75,27.3 71.12,26.67 71.12,22.86 72.39,21.59 72.39,20.32 74.3,18.41 74.3,17.46 v74.93,16.83
N$104  (via drill 0.5)
  Top 0.305: X5.3.1 57.15,24.77 | 57.15,24.77 IC3.4 | IC9.1 50.8,14.61 55.24,14.61 55.88,13.97 55.88,12.7 56.52,12.06 v71.44,12.06 | 57.15,24.77 60.33,24.77 60.96,24.13 60.96,22.86 61.59,22.23 66.04,22.23 IC9.9
  Bottom 0.305: IC11.11 79.7,19.38 78.98,19.38 75.35,15.75 74.42,15.75 73.29,16.88 73.29,18.3 70.64,20.95 IC9.9 67.28,20.93 67.28,20.34 71.44,16.19 v71.44,12.06
N$105  (via drill 0.5)
  Top 0.305: v104.14,48.9 102.55,50.48 75.27,50.48 72.39,53.37 66.17,53.37 65.58,53.95 60.53,53.95 57.38,50.8 39.37,50.8 38.1,49.53 36.2,49.53 33.66,52.07 32.38,52.07 31.75,51.44 31.75,50.8 30.48,49.53 15.3,49.53 11.81,46.04 v4.45,46.04 | v104.14,43.81 104.14,36.2 103.5,35.56 99.69,35.56 99.06,34.92 99.06,33.02 98.74,32.7 93.73,32.7 90.17,29.15 v90.17,28.89 | 122.1 IC4.5
  Bottom 0.305: IC6.13 6.35,12.06 3.17,12.06 2.54,12.7 2.54,44.13 v4.45,46.04 | v104.14,48.9 v104.14,43.81 | 122.1 90.17,26.04 | IC10.4 IC10.3 99.69,13.34 98.42,14.61 95.25,14.61 91.44,18.41 91.44,24.77 90.17,26.04 | 90.17,26.04 v90.17,28.89
N$106  (via drill 0.5)
  Top 0.305: v93.34,22.86 92.71,22.23 78.74,22.23 IC4.3 120.1
  Bottom 0.305: IC10.5 104.14,14.61 99.69,14.61 99.06,15.24 97.79,15.24 96.52,16.51 96.52,21.59 95.89,22.23 93.98,22.23 v93.34,22.86
N$107  (via drill 0.5)
  Top 0.305: IC4.2 119.1 77.47,28.57 86.87,28.57 88.77,26.67 92.01,26.67 94.04,28.7 v108.01,28.7
  Bottom 0.305: IC10.6 107.95,14.61 106.68,15.88 106.68,25.46 108.01,26.8 v108.01,28.7
N$108  (via drill 0.5)
  Top 0.305: IC10.7 110.49,15.24 109.22,16.51 108.58,16.51 107.95,15.88 102.23,15.88 101.6,16.51 101.6,17.14 100.97,17.78 100.08,17.78 98.17,15.88 92.08,15.88 91.44,15.24 v90.17,15.24 | IC4.4 121.1
  Bottom 0.305: v90.17,15.24 90.17,16.51 87.63,19.05 87.63,21.59 87,22.23 81.28,22.23 IC4.4
N$109  (via drill 0.5)
  Top 0.305: v85.09,17.78 96.84,17.78 97.47,18.41 104.84,18.41 v105.47,17.78 | IC10.12 IC10.13
  Bottom 0.305: 126.1 IC5.5 IC10.12 105.41,17.84 v105.47,17.78 | IC11.5 85.09,14.61 v85.09,17.78
N$110  (via drill 0.5)
  Top 0.305: v10.16,6.35 7.3,6.35 1.91,11.75 1.91,32.38 2.54,33.02 4.45,33.02 5.08,33.66 5.08,38.1 3.81,39.37 3.17,39.37 2.54,40.01 2.54,42.55 4.45,44.45 11.18,44.45 15.62,48.9 31.11,48.9 31.75,49.53 34.92,49.53 35.56,48.9 39.37,48.9 40.01,49.53 57.15,49.53 60.96,53.34 65.18,53.34 65.81,52.7 71.12,52.7 74.3,49.53 98.42,49.53 100.97,46.99 106.05,46.99 v107.95,45.09 | IC5.3 101.6,22.23 106.68,22.23 IC10.11
  Bottom 0.305: 124.1 IC5.3 | v10.16,6.35 IC6.12 | IC10.11 109.22,22.23 109.22,34.92 108.58,35.56 107.31,35.56 106.68,36.2 106.68,41.27 107.95,42.55 v107.95,45.09
N$111  (via drill 0.5)
  Top 0.305: v103.13,17.14 103.5,17.14 104.14,16.51 106.68,16.51 107.31,17.14 v107.69,17.14
  Bottom 0.305: 123.1 IC5.2 99.06,22.23 99.06,15.88 99.08,15.85 99.31,15.85 99.92,15.24 101.6,15.24 103.13,16.77 v103.13,17.14 | v107.69,17.14 107.69,18.16 IC10.10
N$112  (via drill 0.5)
  Top 0.305: IC10.1 96.52,12.06 100.97,12.06 101.6,12.7 101.6,15.24 | 101.6,15.24 v100.33,16.51 | 101.6,15.24 v108.84,15.24
  Bottom 0.305: 125.1 IC5.4 101.6,22.23 101.6,17.78 v100.33,16.51 | v108.84,15.24 110.75,15.24 112.02,16.51 112.02,19.05 113.03,20.06 IC10.9
N$113  (via drill 0.5)
  Top 0.305: X5.4.1 60.33,25.4 68.58,25.4 69.22,26.04 71.75,26.04 v72.39,25.4 | v59.44,17.27 58.78,16.61 57.94,16.61 56.87,17.68 48.96,17.68 48.45,17.17 48.28,17.17 48.26,17.14 43.18,17.14 42.99,17.34 v35.56,17.34 | v34.29,8.26 33.02,8.26 32.38,8.89 27.3,8.89 26.04,7.62 17.14,7.62 v16.51,8.26
  Bottom 0.305: IC11.8 88.9,24.13 88.27,24.77 73.03,24.77 v72.39,25.4 | X5.4.1 IC3.5 IC9.12 59.31,20.57 59.31,17.4 v59.44,17.27 | IC6.6 16.51,4.45 v16.51,8.26 15.24,9.53 IC6.10 | IC7.11 v35.56,17.34 35.56,15.24 34.29,13.97 v34.29,8.26
N$114  (via drill 0.5)
  Top 0.305: v45.4,3.17 45.88,2.7 47.78,2.7 50.16,5.08 53.98,5.08 IC12.3 55.56,2.86 57.15,1.27 70.48,1.27 v71.12,1.91
  Bottom 0.305: v71.12,1.91 78.74,1.91 79.38,2.54 79.38,12.7 IC11.3 | IC7.3 31.76,12.07 31.76,6.9 31.75,6.9 31.75,2.54 32.38,1.91 44.13,1.91 v45.4,3.17
N$115
  Bottom 0.305: IC7.5 38.1,13.02 36.83,11.75 36.83,7.62 33.02,3.81 IC13.3
N$116  (via drill 0.5)
  Top 0.305: v71.44,17.78 68.26,17.78 67.94,18.1 64.33,18.1 63.12,16.89 60.54,16.89 59.66,16 57.69,16 56.62,17.07 49.45,17.07 48.9,16.51 43.18,16.51 41.72,15.05 36.28,15.05 35.8,15.53 30.19,15.53 29.79,15.93 28.63,15.93 27.94,15.24 IC7.1
  Bottom 0.305: v71.44,17.78 71.44,17.46 73.66,15.24 IC11.1
N$117
  Bottom 0.305: IC13.1 23.5,3.17 22.23,4.45 22.23,8.89 IC6.8
N$118  (via drill 0.5)
  Top 0.305: v39.37,16.26 34.04,16.26 v33.02,17.27
  Bottom 0.305: IC13.10 38.1,11.43 39.37,12.7 v39.37,16.26 | IC7.12 v33.02,17.27
N$119
  Bottom 0.305: IC13.9 IC13.6
N$120
  Bottom 0.305: IC13.4 39.37,6.99 39.37,11.75 40.64,13.02 IC7.6
N$121  (via drill 0.5)
  Top 0.305: v41.91,6.99 41.34,6.41 31.05,6.41 v30.54,6.92
  Bottom 0.305: IC13.13 30.54,10.73 v30.54,6.92 | v41.91,6.99 43.18,8.26 IC13.8
N$122  (via drill 0.5)
  Top 0.305: IC8.2 6.99,13.97 6.99,16.51 8.26,17.78 17.14,17.78 19.68,15.24 20.95,15.24 21.59,15.88 26.23,15.88 v26.73,15.37 | v24.77,27.94 27.3,27.94 27.94,28.57 38.42,28.57 40.45,26.54 44.77,26.54 v45.4,27.18
  Bottom 0.305: IC8.2 5.71,13.34 3.81,15.24 3.81,17.78 5.71,19.68 7.62,19.68 IC8.14 | IC12.11 57.15,12.06 53.98,12.06 53.34,12.7 53.34,17.78 55.88,20.32 55.88,22.23 | v26.73,15.37 26.73,19.94 25.4,21.27 25.4,27.3 v24.77,27.94 | v45.4,27.18 46.16,27.18 48.2,29.21 54.61,29.21 55.88,27.94 55.88,22.23 | IC9.15 53.34,22.23 55.88,22.23
N$123  (via drill 0.5)
  Top 0.305: v75.88,18.1 74.93,19.05 71.12,19.05 70.48,18.41 68.58,18.41 68.26,18.73 63.06,18.73 v62.23,17.91 | IC12.2 51.44,1.27 23.75,1.27 v22.48,2.54
  Bottom 0.305: IC11.13 76.2,18.41 v75.88,18.1 | IC12.2 53.98,3.17 55.88,5.08 55.88,6.99 56.52,7.62 57.15,7.62 59.69,10.16 59.69,11.43 60.94,12.68 60.94,14.33 62.23,15.62 v62.23,17.91 | v22.48,2.54 22.48,3.17 21.08,4.57 19.18,4.57 19.05,4.45 17.78,5.71 IC6.9
N$124  (via drill 0.5)
  Top 0.305: v49.53,6.35 50.8,7.62 58.74,7.62 60.64,5.71 68.26,5.71 68.9,6.35 82.11,6.35 v82.61,6.86
  Bottom 0.305: IC12.1 50.8,5.08 v49.53,6.35 | v82.61,6.86 82.55,6.92 82.55,15.24 83.82,16.51 IC11.10
N$125  (via drill 0.5)
  Top 0.305: v66.04,7.37 66.29,7.62 71.75,7.62 v72.39,8.26 | v79.38,17.78 80.64,19.05 91.44,19.05 92.08,18.41 96.52,18.41 97.16,19.05 108.58,19.05 v110.17,17.46 111.76,15.88 111.76,12.06 111.12,11.43 111.12,5.08 X8.4.1
  Bottom 0.305: IC12.9 66.04,8.26 v66.04,7.37 | v72.39,8.26 73.66,8.26 74.93,9.53 74.93,13.97 78.74,17.78 v79.38,17.78 | v110.17,17.46 110.17,18.73 111.76,20.32 111.76,31.75 112.39,32.38 113.03,32.38 114.3,33.66 114.3,38.1 113.03,39.37 112.39,39.37 111.76,40.01 111.76,45.09 X3.2.1
N$126  (via drill 0.5)
  Top 0.305: v31,16.54 27.57,16.54 27.56,16.54 20.34,16.54 v20.32,16.51
  Bottom 0.305: 112.1 IC2.3 31.75,17.14 31.11,16.51 31.03,16.51 v31,16.54 | IC8.11 16.51,20.32 13.97,17.78 X6.3.1 14.61,15.88 15.88,14.61 18.41,14.61 v20.32,16.51
N$127  (via drill 0.5)
  Top 0.305: X4.4.1 16.51,27.56 | v43.5,15.24 44.13,15.88 48.9,15.88 48.92,15.9 49.15,15.9 49.71,16.46 56.37,16.46 57.59,15.24 60.33,15.24 v60.96,15.88 64.2,15.88 v65.15,16.83 | IC11.12 77.47,22.23 v70.17,22.23 | 16.51,27.56 17.53,28.57 20,28.57 21.27,27.3 22.54,27.3 v23.18,27.94 | v24.13,22.86 26.04,24.77 37.47,24.77 38.1,24.13 IC7.10 | Q1.G 32.38,43.18 31.75,43.81 31.75,47.62 31.11,48.26 15.88,48.26 10.16,42.55 10.16,33.66 8.89,32.38 3.17,32.38 2.54,31.75 2.54,29.84 4.83,27.56 16.51,27.56
  Bottom 0.305: IC9.3 57.15,15.88 v60.96,15.88 | v43.5,15.24 38.1,20.64 IC7.10 | v70.17,22.23 68.58,23.81 68.58,24.13 67.94,24.77 64.14,24.77 63.5,24.13 63.5,20.38 65.15,18.73 v65.15,16.83 | v23.18,27.94 22.86,27.62 22.86,24.13 v24.13,22.86
N$128  (via drill 0.5)
  Top 0.305: IC8.15 6.35,19.68 6.99,19.05 22.23,19.05 22.86,18.41 25.81,18.41 26.35,18.96 45.4,18.96 45.95,18.41 47.62,18.41 48.17,18.96 60.07,18.96 v60.58,18.45
  Bottom 0.305: IC12.8 65.41,10.79 63.5,12.7 63.5,15.01 63.45,15.07 63.45,18.3 62.76,19 61.12,19 v60.58,18.45
N$129  (via drill 0.5)
  Top 0.305: IC11.6 85.09,12.06 73.03,12.06 71.75,10.79 71.75,9.53 70.48,8.26 68.58,8.26 67.94,8.89 51.44,8.89 51.41,8.87 49.28,8.87 48.67,8.26 40.64,8.26 39.5,7.11 32.26,7.11 31.11,8.26 27.94,8.26 26.67,6.99 v12.7,6.99
  Bottom 0.305: IC6.11 v12.7,6.99
N$131  (via drill 0.5)
  Top 0.305: v49.53,42.23 56.52,42.23 56.83,41.91 59.63,41.91 59.88,41.66 v65.6,41.66
  Bottom 0.305: IC13.11 35.56,11.43 36.83,12.7 36.83,21.59 38.1,22.86 38.1,24.13 40.64,26.67 43.18,26.67 44.32,27.81 44.32,29.08 48.26,33.02 48.26,38.42 49.53,39.69 v49.53,42.23 | RN9.5 66.61,37.47 65.6,38.48 v65.6,41.66
N$132  (via drill 0.5)
  Top 0.305: IC12.12 54.61,12.06 48.58,12.06 v48.26,11.75 | v48.9,27.3 50.8,29.21 66.36,29.21 v66.99,28.57 | v68.58,51.44 67.94,52.07 65.59,52.07 64.95,52.7 62.87,52.7 C14.1
  Bottom 0.305: v48.9,27.3 48.9,25.4 48.26,24.77 v48.26,11.75 | v66.99,28.57 66.04,29.53 66.04,34.92 67.31,36.2 68.58,36.2 RN9.6 71.12,38.73 71.12,41.27 70.48,41.91 69.85,41.91 68.58,43.18 68.58,45.09 69.85,46.35 69.85,50.16 v68.58,51.44
N$133
  Top 0.305: RN16.5 X7.1.1
  Bottom 0.305: RN7.2 98.42,9.53 98.42,7.62 X7.1.1 | S2.3 80.92,5.88 83.5,3.3 83.5,2.54 84.77,1.27 95.25,1.27 RN16.5
N$134  (via drill 0.5)
  Top 0.305: v54.86,5.97 55.24,5.97 57.15,4.06 57.15,2.54 57.78,1.91 69.53,1.91 70.8,3.17 71.44,3.17 72.39,2.22 86.68,2.22 v87,2.54 88.27,1.27 107.95,1.27 109.73,3.05 109.73,7.49 v109.09,8.13 | v113.03,18.41 113.03,18.6 114.25,19.82 114.25,22.17 114.3,22.23 v114.3,27.94 | v115.02,31.67 114.3,32.39 114.3,41.91 112.39,43.81 107.31,43.81 104.78,46.35 100.33,46.35 98.42,48.26 69.85,48.26 66.67,51.44 C15.1
  Bottom 0.305: RN7.1 92.71,6.35 87.63,6.35 87,5.71 v87,2.54 | v54.86,5.97 53.34,7.49 IC12.13 | v109.09,8.13 111.12,10.16 111.12,11.43 111.76,12.06 111.76,13.97 113.03,15.24 v113.03,18.41 | v114.3,27.94 114.3,31.11 114.94,31.75 v115.02,31.67
N$135
  Bottom 0.305: RN9.4 64.14,38.1 64.14,38.73 | 64.14,38.73 C17.1 | 64.14,38.73 61.59,38.73 60.96,38.1 60.96,27.3 61.59,26.67 61.59,25.4 60.96,24.77 60.96,20.32 61.59,19.68 63.12,19.68 64.14,18.67 64.14,16.51 64.14,16.41 64.73,15.82 64.83,15.82 66.04,14.61 66.04,12.7 67.31,11.43 67.31,6.99 66.04,5.71 63.34,5.71 62.23,6.82 62.23,7.62 61.59,8.26 60.33,8.26 59.69,7.62 59.69,5.71 60.96,4.45 IC12.5
N$136  (via drill 0.5)
  Top 0.305: IC7.8 44.45,22.23 50.16,22.23 50.8,22.86 50.8,25.44 50.75,25.49 50.75,26.75 51.94,27.94 63.5,27.94 v64.14,27.3
  Bottom 0.305: v64.14,27.3 63.5,27.94 63.5,36.2 RN9.3
N$137
  Top 0.305: S3.1 89.06,3.65 90.81,1.91 98.42,1.91 RN16.4 X7.2.1
  Bottom 0.305: RN7.3 100.33,8.89 X7.2.1
N$138  (via drill 0.5)
  Top 0.305: IC12.4 60.33,5.08 68.58,5.08 69.22,5.71 v93.98,5.71 | C16.1 15.62,50.8 11.81,46.99 5.71,46.99 v3.81,48.9
  Bottom 0.305: v93.98,5.71 97.79,9.53 97.79,10.79 98.42,11.43 102.87,11.43 RN7.4 | IC12.4 56.52,1.27 5.08,1.27 1.91,4.45 1.91,46.99 v3.81,48.9
N$139  (via drill 0.5)
  Top 0.305: v63.5,6.99 64.14,6.35 67.31,6.35 67.94,6.99 76.83,6.99 77.85,8 85.09,8 85.47,7.62 v87,7.62 | v96.52,45.72 80.64,45.72 79.38,46.99 v67.94,46.99
  Bottom 0.305: IC12.10 63.5,8.26 v63.5,6.99 | v67.94,46.99 67.31,46.35 67.31,45.09 65.41,43.18 64.77,43.18 C18.1 | v96.52,45.72 96.52,30.36 98.31,28.57 102.87,28.57 104.14,27.3 104.14,17.14 106.68,14.61 106.68,12.06 106.63,12.12 | v87,7.62 92.71,7.62 94.61,9.53 94.61,10.79 95.94,12.12 106.63,12.12 | 106.63,12.12 108.53,12.12 109.22,11.43 RN7.6
N$140
  Top 0.305: 102.87,8.89 X7.3.1 RN16.3 | RN7.5 105.41,8.89 102.87,8.89 | 102.87,8.89 77.15,8.89 75.81,10.24 S1.3
N$143
  Bottom 0.305: IC8.1 3.17,13.97 3.17,18.41 5.08,20.32 5.08,24.13 6.99,26.04 X4.1.1
N$144
  Top 0.305: IC9.7 66.04,14.61 67.94,14.61 69.22,13.34 71.12,13.34 73.03,15.24 86.36,15.24 87.63,13.97 87.63,12.7 88.58,11.75 95.89,11.75 96.2,11.43 107.31,11.43 107.95,10.79 107.95,9.53 X7.4.1
N$145  (via drill 0.5)
  Top 0.305: IC8.3 10.16,14.61 22.23,14.61 24.13,12.7 v25.08,12.7 | v27.94,6.35 28.57,5.71 v43.81,5.71 | v45.09,10.79 48.9,14.61 49.94,14.61 50.57,15.24 55.56,15.24 57.15,13.65 IC9.4
  Bottom 0.305: v25.08,12.7 26.67,11.11 26.67,7.62 v27.94,6.35 | v43.81,5.71 45.09,6.99 v45.09,10.79
V+  (via drill 0.5)
  Top 0.305: IC1.16 5.08,29.84 C2.2 25.4,29.84 IC2.16 27.94,29.84 C3.2 | IC3.16 50.8,29.84 58.42,29.84 | IC4.16 73.66,29.84 | C1.2 96.52,29.84 IC5.16 93.98,29.84 C5.2 90.68,27.81 89.53,27.81 87.5,29.84 73.66,29.84 | IC8.16 5.08,22.23 6.99,22.23 7.62,21.59 7.62,20.32 8.26,19.68 C7.2 25.4,19.68 26.67,20.95 IC7.14 29.21,19.68 C12.2 48.26,19.68 IC9.16 50.8,19.68 C11.2 71.12,19.68 72.39,20.95 IC11.14 74.93,19.68 C10.2 93.98,20.95 IC10.16 | IC6.14 6.35,9.53 C9.2 26.67,9.53 IC13.14 29.21,9.53 C13.2 48.26,9.53 49.53,10.79 IC12.14 52.07,9.53 C8.2 | RN1.1 58.42,33.02 58.42,29.84 | IC3.16 48.26,29.84 C3.2 | v12.7,42.55 13.34,42.55 17.14,46.35 26.99,46.35 v27.62,45.72 | IC6.1 6.35,1.91 13.97,1.91 IC6.5 | IC10.16 IC5.1 | 73.66,29.84 73.66,26.63 73.61,26.58 73.61,24.71 IC4.1 | C3.2 46.99,26.67 45.72,25.4 45.72,24.13 46.35,23.5 IC3.1 | IC3.16 48.26,32.38 48.26,38.1 47.6,38.76 40.64,38.76 39.37,37.49 RN5.1 | C6.2 115.57,19.28 113.55,17.26 112.66,17.26 110.24,19.68 96.52,19.68 IC10.16 | C4.2 58.42,29.84
  Top 0.61: v115.57,47.62 111.76,51.44 X3.1.1
  Bottom 0.305: Q1.S 27.94,43.18 27.94,45.72 | 27.94,45.72 27.94,50.8 29.21,52.07 37.78,52.07 39.37,50.48 RN5.1 | IC4.16 71.12,29.84 C4.2 | v27.62,45.72 27.94,45.72 | v12.7,42.55 12.7,29.21 11.05,27.56 3.81,27.56 | IC1.16 3.81,27.56 | IC4.1 72.39,22.54 73.66,21.27 IC11.14 | IC6.14 IC6.1 | IC3.1 IC9.16 49.53,15.24 50.8,13.97 IC12.14 | IC8.16 IC1.1 3.81,27.56 | IC7.14 27.94,21.27 26.67,22.54 IC2.1 26.67,27.47 24.29,29.84 C2.2 | X8.3.1 111.12,3.81 RN16.1 | IC5.1 94.61,24.13 94.61,30.48 IC5.16 | C7.2 25.4,18.41 25.4,13.97 27.94,11.43 IC13.14
  Bottom 0.61: X8.3.1 117.47,10.16 117.47,19.68 | 117.47,19.68 117.47,27.94 C1.2 117.47,31.75 117.47,45.72 v115.57,47.62 | 117.47,19.68 C6.2

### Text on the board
tPlace: GND | DISP | V+ | V 1.1 | IN | TAG | MONAT | JAHR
